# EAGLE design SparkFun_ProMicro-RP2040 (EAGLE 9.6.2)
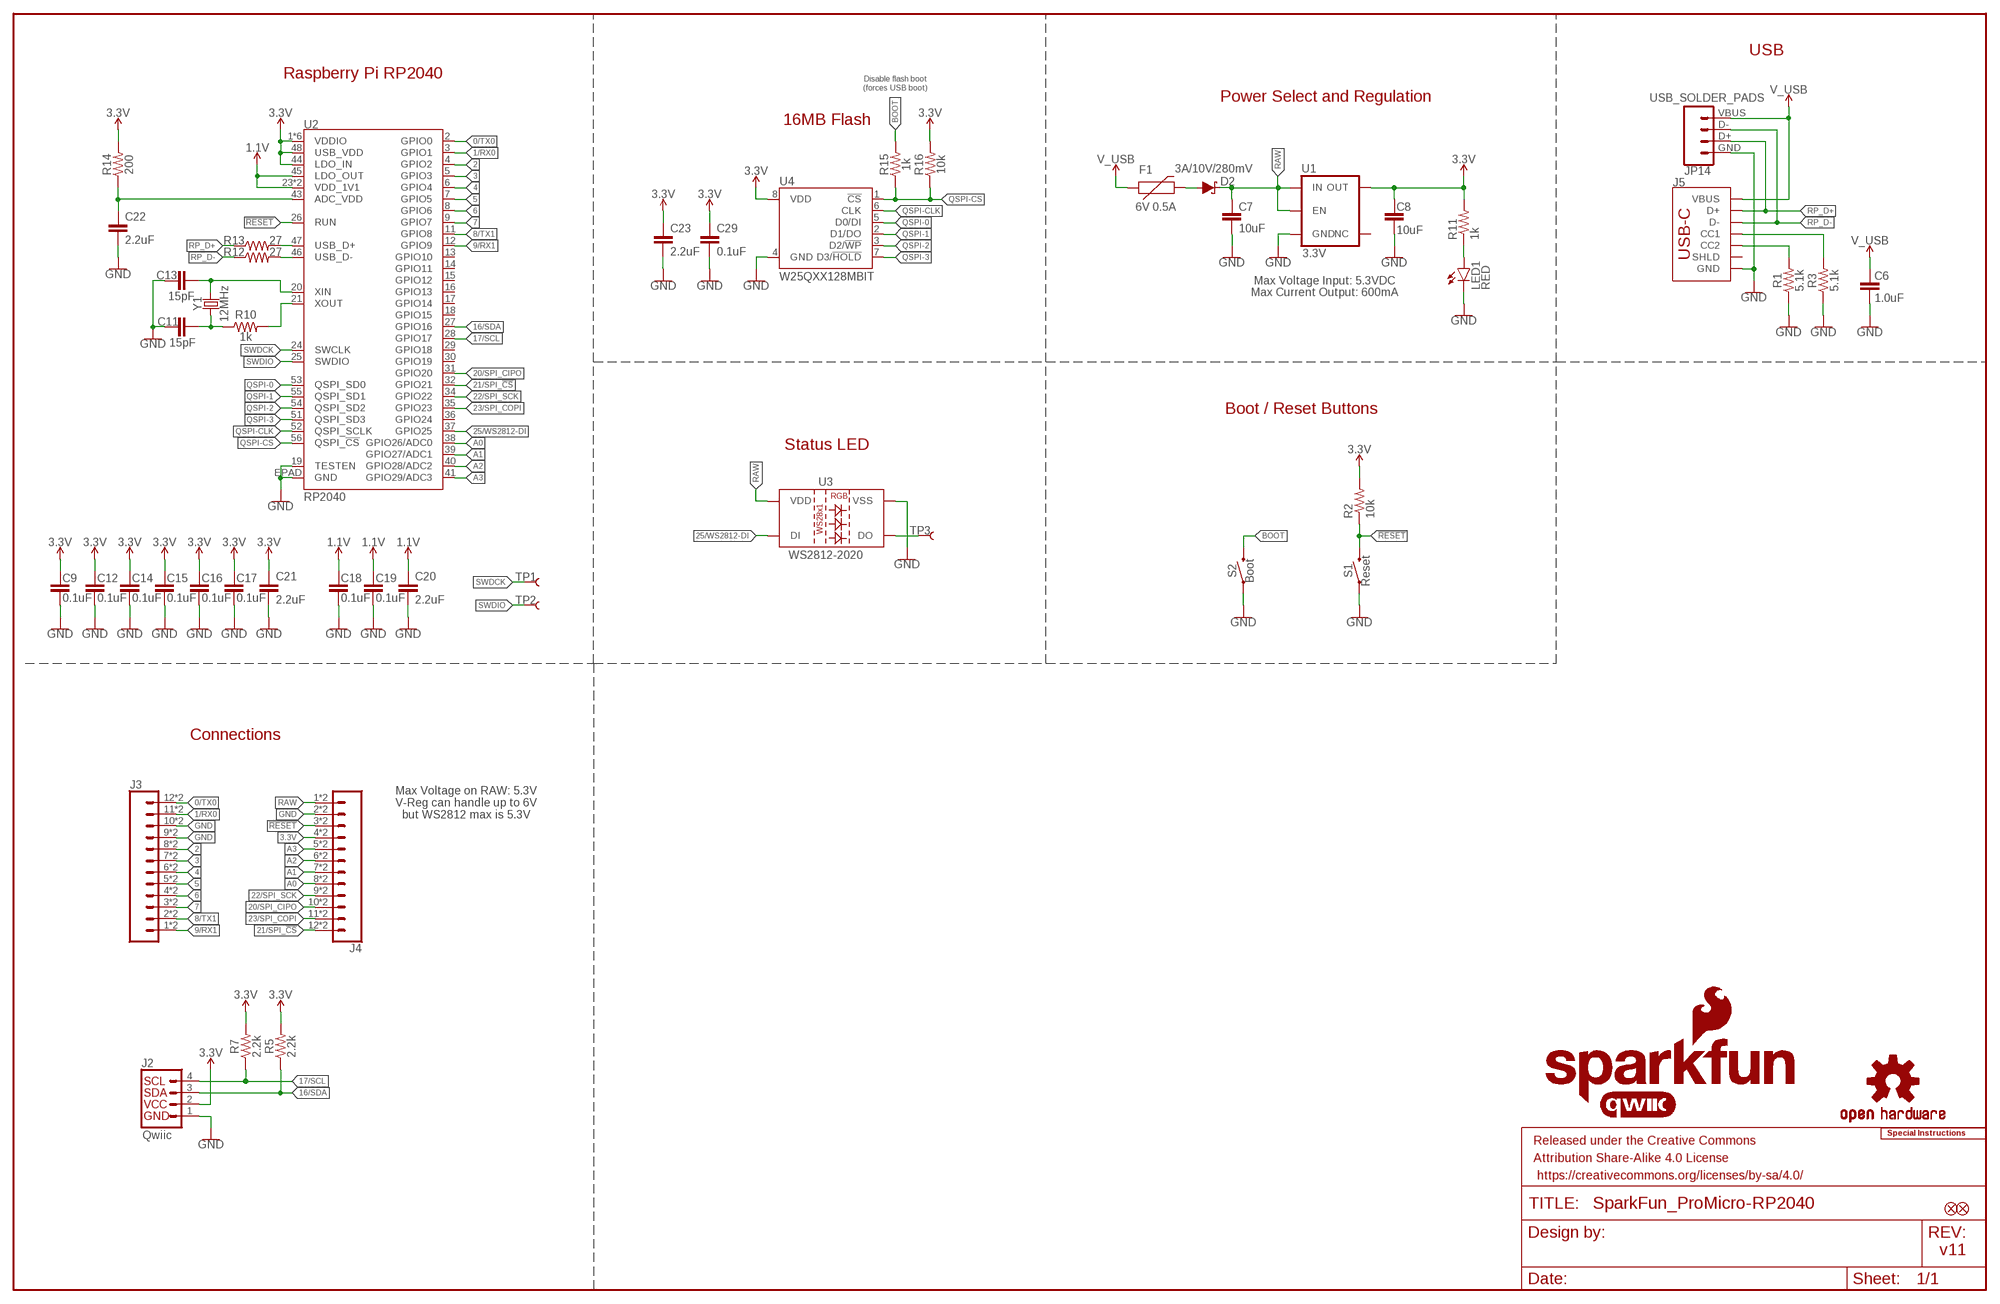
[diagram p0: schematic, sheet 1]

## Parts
C6  1.0uF  1.0UF-0402T-16V-10%  [0402-TIGHT]
C7  10uF  10UF-0402T-6.3V-20%  [0402-TIGHT]
C8  10uF  10UF-0402T-6.3V-20%  [0402-TIGHT]
C9  0.1uF  0.1UF-0402T-6.3V-10%-X7R  [0402-TIGHT]
C11  15pF  15PF-0402T-50V-5%  [0402-TIGHT]
C12  0.1uF  0.1UF-0402T-6.3V-10%-X7R  [0402-TIGHT]
C13  15pF  15PF-0402T-50V-5%  [0402-TIGHT]
C14  0.1uF  0.1UF-0402T-6.3V-10%-X7R  [0402-TIGHT]
C15  0.1uF  0.1UF-0402T-6.3V-10%-X7R  [0402-TIGHT]
C16  0.1uF  0.1UF-0402T-6.3V-10%-X7R  [0402-TIGHT]
C17  0.1uF  0.1UF-0402T-6.3V-10%-X7R  [0402-TIGHT]
C18  0.1uF  0.1UF-0402T-6.3V-10%-X7R  [0402-TIGHT]
C19  0.1uF  0.1UF-0402T-6.3V-10%-X7R  [0402-TIGHT]
C20  2.2uF  2.2UF-0402_TIGHT-10V-10%-X5R  [0402-TIGHT]
C21  2.2uF  2.2UF-0402_TIGHT-10V-10%-X5R  [0402-TIGHT]
C22  2.2uF  2.2UF-0402_TIGHT-10V-10%-X5R  [0402-TIGHT]
C23  2.2uF  2.2UF-0402_TIGHT-10V-10%-X5R  [0402-TIGHT]
C29  0.1uF  0.1UF-0402T-6.3V-10%-X7R  [0402-TIGHT]
D2  3A/10V/280mV  DIODE-SCHOTTKY-BAT60A  [SOD-323]
F1  6V 0.5A  PPTC_6V500MA  [0805]
FRAME2  FRAME-LEDGER  [CREATIVE_COMMONS]
J2  Qwiic  QWIIC_CONNECTORJS-1MM  [JST04_1MM_RA]
J3  CONN_12CASTLE  [1X12_CASTELLATED]
J4  CONN_12CASTLE  [1X12_CASTELLATED]
J5  USB Female Type C Connector  USB_C_4-LAYER_PADS  [USB-C-16P_4LAYER-PADS]
JP1  FIDUCIAL1X2  [FIDUCIAL-1X2]
JP2  FIDUCIAL1X2  [FIDUCIAL-1X2]
JP14  USB_SOLDER_PADS  [USB-SOLDER-PADS]
LED1  RED  LED-RED0603  [LED-0603]
LOGO1  SFE_LOGO_NAME_FLAME.1_INCH  [SFE_LOGO_NAME_FLAME_.1]
LOGO3  QWIIC_LOGO_6MM  [QWIIC_6MM]
LOGO4  SFE_LOGO_FLAME.1_INCH  [SFE_LOGO_FLAME_.1]
LOGO5  SPECIAL_INSTRUCTIONS-ORDERING  [ORDERING_INSTRUCTIONS]
R1  5.1k  5.1KOHM-0402T-1/16W-1%  [0402-TIGHT]
R2  10k  10KOHM-0402T-1/16W-1%  [0402-TIGHT]
R3  5.1k  5.1KOHM-0402T-1/16W-1%  [0402-TIGHT]
R5  2.2k  2.2KOHM-0402T-1/16W-1%  [0402-TIGHT]
R7  2.2k  2.2KOHM-0402T-1/16W-1%  [0402-TIGHT]
R10  1k  1KOHM-0402T-1/16W-1%  [0402-TIGHT]
R11  1k  1KOHM-0402T-1/16W-1%  [0402-TIGHT]
R12  27  27OHM  [0402-TIGHT]
R13  27  27OHM  [0402-TIGHT]
R14  200  200OHM-0402T-1/16W-1%  [0402-TIGHT]
R15  1k  1KOHM-0402T-1/16W-1%  [0402-TIGHT]
R16  10k  10KOHM-0402T-1/16W-1%  [0402-TIGHT]
S1  Reset  MOMENTARY-SWITCH-SPST-SMD-4.6X2.8MM  [TACTILE_SWITCH_SMD_4.6X2.8MM]
S2  Boot  MOMENTARY-SWITCH-SPST-SMD-4.6X2.8MM  [TACTILE_SWITCH_SMD_4.6X2.8MM]
TP1  TEST-POINT3X5  [PAD.03X.05]
TP2  TEST-POINT3X5  [PAD.03X.05]
TP3  TEST-POINT3X5  [PAD.03X.05]
U1  3.3V  V_REG_AP2112K-3.3V  [SOT23-5]
U2  RP2040  [QFN-56]
U3  WS2812-2020  [WS2812-2020]
U4  W25QXX128MBIT  W25QXX128MBIT-6X5-SKINNY_CENTER  [WSON-8-6X5-SKINNY_CENTERPAD]
U$3  OSHW-LOGOMINI  [OSHW-LOGO-MINI]
Y1  12MHz  CRYSTAL-12MHZ  [CRYSTAL-SMD-2X2.5MM]

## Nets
0/TX0: J3.12 J3.12B U2.2(GPIO0)
1.1V: C18.1 C19.1 C20.1 U2.23(VDD_1V1) U2.45(LDO_OUT) U2.50(VDD_1V1)
1/RX0: J3.11 J3.11B U2.3(GPIO1)
2: J3.8 J3.8B U2.4(GPIO2)
3: J3.7 J3.7B U2.5(GPIO3)
3.3V: C8.2 C9.1 C12.1 C14.1 C15.1 C16.1 C17.1 C21.1 C23.1 C29.1 J2.2 J4.4 J4.4B R2.2 R5.2 R7.2 R11.2 R14.2 R16.2 U1.5(OUT) U2.1(VDDIO) U2.10(VDDIO) U2.22(VDDIO) U2.33(VDDIO) U2.42(VDDIO) U2.44(LDO_IN) U2.48(USB_VDD) U2.49(VDDIO) U4.8(VDD)
4: J3.6 J3.6B U2.6(GPIO4)
5: J3.5 J3.5B U2.7(GPIO5)
6: J3.4 J3.4B U2.8(GPIO6)
7: J3.3 J3.3B U2.9(GPIO7)
8/TX1: J3.2 J3.2B U2.11(GPIO8)
9/RX1: J3.1 J3.1B U2.12(GPIO9)
16/SDA: J2.3 R5.1 U2.27(GPIO16)
17/SCL: J2.4 R7.1 U2.28(GPIO17)
20/SPI_CIPO: J4.10 J4.10B U2.31(GPIO20)
21/SPI_!CS!: J4.12 J4.12B U2.32(GPIO21)
22/SPI_SCK: J4.9 J4.9B U2.34(GPIO22)
23/SPI_COPI: J4.11 J4.11B U2.35(GPIO23)
25/WS2812-DI: U2.37(GPIO25) U3.3(DI)
!RESET!: J4.3 J4.3B R2.1 S1.3 S1.4 U2.26(RUN)
A0: J4.8 J4.8B U2.38(GPIO26/ADC0)
A1: J4.7 J4.7B U2.39(GPIO27/ADC1)
A2: J4.6 J4.6B U2.40(GPIO28/ADC2)
A3: J4.5 J4.5B U2.41(GPIO29/ADC3)
ADC_VDD: C22.1 R14.1 U2.43(ADC_VDD)
BOOT: R15.2 S2.3 S2.4
GND: C6.1 C7.1 C8.1 C9.2 C11.1 C12.2 C13.1 C14.2 C15.2 C16.2 C17.2 C18.2 C19.2 C20.2 C21.2 C22.2 C23.2 C29.2 J2.1 J3.9 J3.9B J3.10 J3.10B J4.2 J4.2B J5.GND J5.GND2(GND) JP14.GND LED1.C R1.1 R3.1 S1.1 S1.2 S2.1 S2.2 U1.2(GND) U2.19(TESTEN) U2.EPAD(GND) U3.2(VSS) U4.4(GND)
N$1: TP3.P$1 U3.1(DO)
N$9: J5.A5(CC1) R3.2
N$10: J5.B5(CC2) R1.2
N$38: LED1.A R11.1
QSPI-0: U2.53(QSPI_SD0) U4.5(D0/DI)
QSPI-1: U2.55(QSPI_SD1) U4.2(D1/DO)
QSPI-2: U2.54(QSPI_SD2) U4.3(D2/!WP!)
QSPI-3: U2.51(QSPI_SD3) U4.7(D3/!HOLD!)
QSPI-CLK: U2.52(QSPI_SCLK) U4.6(CLK)
QSPI-CS: R15.1 R16.1 U2.56(QSPI_!CS!) U4.1(!CS!)
RAW [Power]: C7.2 D2.C J4.1 J4.1B U1.1(IN) U1.3(EN) U3.4(VDD)
RP_D1+: R13.2 U2.47(USB_D+)
RP_D1-: R12.2 U2.46(USB_D-)
RP_D+: J5.A6(D+) J5.B6(D+) JP14.D+ R13.1
RP_D-: J5.A7(D-) J5.B7(D-) JP14.D- R12.1
SWDCK: TP1.P$1 U2.24(SWCLK)
SWDIO: TP2.P$1 U2.25(SWDIO)
USB_RAW [Power]: D2.A F1.2
V_USB [Power]: C6.2 F1.1 J5.VBUS1(VBUS) J5.VBUS2(VBUS) JP14.VBUS
X1A: R10.2 U2.21(XOUT)
X1B: C11.2 R10.1 Y1.P1
X2: C13.2 U2.20(XIN) Y1.P3
Unconnected: J5.SHLD1(SHLD) J5.SHLD2(SHLD) J5.SHLD3(SHLD) J5.SHLD4(SHLD) U1.4(NC) U2.13(GPIO10) U2.14(GPIO11) U2.15(GPIO12) U2.16(GPIO13) U2.17(GPIO14) U2.18(GPIO15) U2.29(GPIO18) U2.30(GPIO19) U2.36(GPIO24)

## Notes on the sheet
- USB
- Raspberry Pi RP2040
- Disable flash boot
  (forces USB boot)
- Power Select and Regulation
- 16MB Flash
- Max Voltage Input: 5.3VDC
- Max Current Output: 600mA
- Boot / Reset Buttons
- Status LED
- Connections
- Max Voltage on RAW: 5.3V
  V-Reg can handle up to 6V
  but WS2812 max is 5.3V
- v11

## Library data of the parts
C6 = SparkFun-Capacitors:1.0UF: 1µF ceramic capacitors; PROD_ID: CAP-12417
C7 C8 = SparkFun-Capacitors:10UF: 10.0µF ceramic capacitors; PROD_ID: CAP-14848
C9 C12 C14-C19 C29 = SparkFun-Capacitors:0.1UF: 0.1µF ceramic capacitors; PROD_ID: CAP-14993
C11 C13 = SparkFun-Capacitors:15PF: 15pF ceramic capacitors; PROD_ID: CAP-13063
C20-C23 = SparkFun-Capacitors:2.2UF: 2.2µF ceramic capacitors; PROD_ID: CAP-14232
D2 = SparkFun-DiscreteSemi:DIODE-SCHOTTKY: Schottky diode; PROD_ID: DIO-14072
F1 = SparkFun-Fuses:PPTC: Resettable Fuse PPTC; PROD_ID: RES-13945
FRAME2 = SparkFun-Aesthetics:FRAME-LEDGER: Schematic Frame - Ledger
J2 = SparkFun-Connectors:QWIIC_CONNECTOR: SparkFun I2C Standard Qwiic Connector An SMD 1mm pitch JST connector makes it easy and quick (get it? Qwiic?) to connect I2C devices to each other. The Qwiic system enables fast and solderless connection between popular platforms and various sensors and actuators. We carry 200mm, 100mm, 50mm, and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; PROD_ID: CONN-13694; VALUE: QWIIC_RIGHT_ANGLE
J3 J4 = Castellated:CONN_12: Multi connection point. Often used as Generic Header-pin footprint for 0.1 inch spaced/style header connections On any of the 0.1 inch spaced packages, you can populate with these: Break Away Headers - Straight (PRT-00116) Break Away Male Headers - Right Angle (PRT-00553) Female Headers (PRT-00115)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
J5 = SparkFun-Connectors:USB_C: USB Type C 16Pin Connector Super Speed pins not available on the 16-pin purely SMD connector so this part is best for USB 2.0 implementations. D1 and D2 are tied together enabling D+/- no matter which way the cable is plugged into the connector. The two channel configuration pins (CC1/2) are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; PROD_ID: CONN-14122
JP1 JP2 = SparkFun-Aesthetics:FIDUCIAL: Fiducial Alignment Points
JP14 = SparkFun-Connectors:USB_SOLDER_PADS: Solder pad access to USB pins. Helpful to expose on PCBs so user can attach external USB connector if necessary.
LED1 = SparkFun-LED:LED-RED: Red SMD LED; PROD_ID: DIO-00819
LOGO1 = SparkFun-Aesthetics:SFE_LOGO_NAME_FLAME: SparkFun Font Logo w/ Flame
LOGO3 = SparkFun-Aesthetics:QWIIC_LOGO: Qwiic Logos for placement on schematic and PCB. The 5.5mm silk logo is best for placing next to Qwiic connector.
LOGO4 = SparkFun-Aesthetics:SFE_LOGO_FLAME: SparkFun Flame Logo
LOGO5 = SparkFun-Aesthetics:SPECIAL_INSTRUCTIONS: Special Ordering/Production Instructions Alert
R1 R3 = SparkFun-Resistors:5.1KOHM; PROD_ID: RES-14340
R2 R16 = SparkFun-Resistors:10KOHM: 10kΩ resistor; PROD_ID: RES-14241
R5 R7 = SparkFun-Resistors:2.2KOHM: 2.2kΩ resistor; PROD_ID: RES-14341
R10 R11 R15 = SparkFun-Resistors:1KOHM: 1kΩ resistor; PROD_ID: RES-14342
R12 R13 = SparkFun-Resistors:27OHM: 27Ω resistor; PROD_ID: RES-15238
R14 = SparkFun-Resistors:200OHM: 200Ω resistor; PROD_ID: RES-15550
S1 S2 = SparkFun-Switches:MOMENTARY-SWITCH-SPST: Momentary Switch (Pushbutton) - SPST; PROD_ID: SWCH-15606
TP1-TP3 = SparkFun-Connectors:TEST-POINT: SparkFun Test Points
U1 = SparkFun-IC-Power:V_REG_AP2112: AP2112 - 600mA CMOS LDO Regulator w/ Enable The AP2112 is CMOS process low dropout linear regulator with enable function, the regulator delivers a guaranteed 600mA (min.) continuous load current. Features Output Voltage Accuracy: ±1.5% Output Current: 600mA (Min.) Foldback Short Current Protection: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; PROD_ID: VREG-12457
U2 = RP2040:RP2040: Raspberry Pi RP2040 MCU 56-pin 32-bit Microcontroller with 264kB of SRAM and external flash support up to 16MB Getting Started with the RP2040 Dual-core ARM Cortex M0+ processor, flexible clock running up to 133 MHz 264kB of SRAM, and QSPI control of common flash memory USB 1.1 Host and Device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; PROD_ID: IC-15502
U3 = SparkFun-LED:WS2812-2020; PROD_ID: DIO-15591
U4 = SparkFun-IC-Memory:W25QXX; PROD_ID: IC-15107
U$3 = SparkFun-Aesthetics:OSHW-LOGO: Open-Source Hardware (OSHW) Logo
Y1 = SparkFun-Clocks:CRYSTAL-12MHZ: 12.0MHz Crystal; PROD_ID: XTAL-15540

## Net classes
1 Power: width 0.127 mm, clearance 0.178 mm

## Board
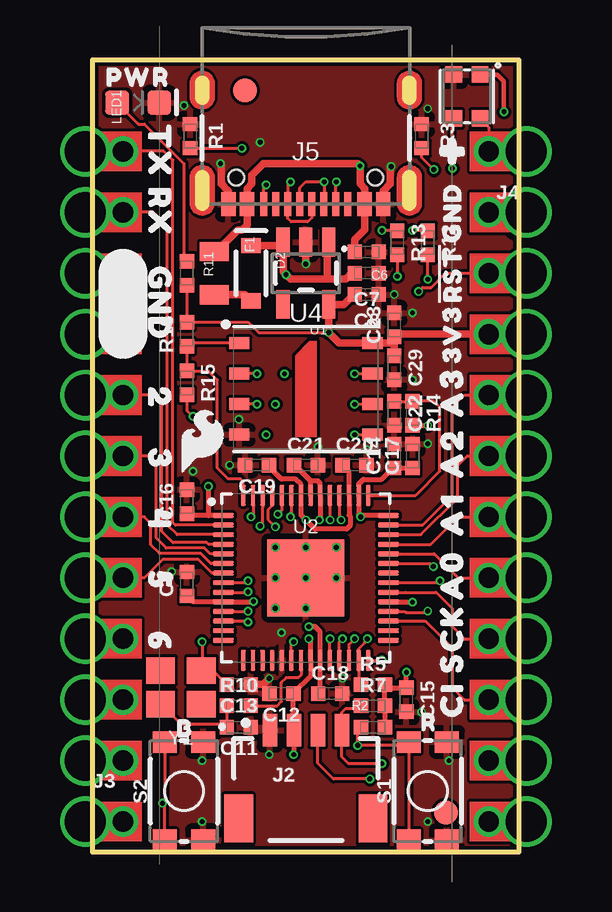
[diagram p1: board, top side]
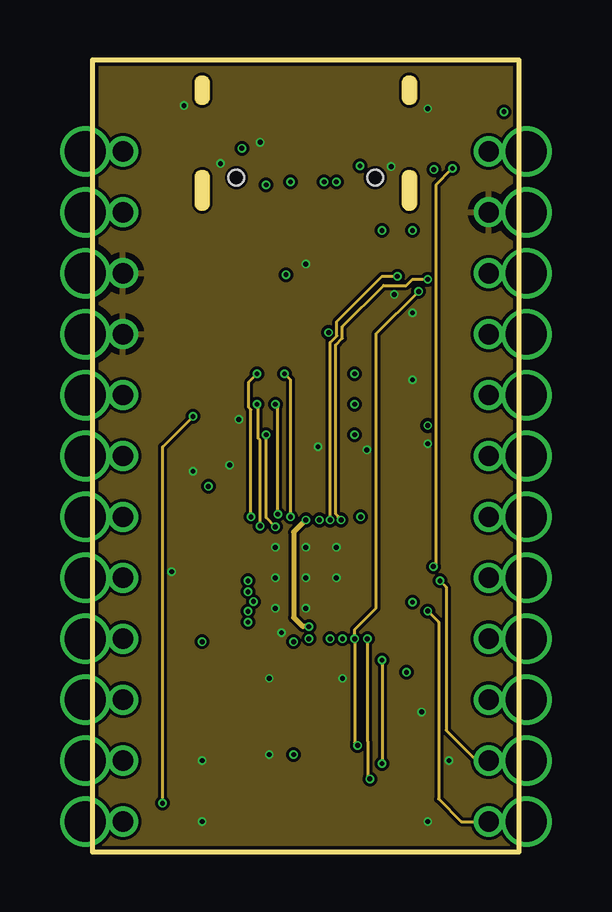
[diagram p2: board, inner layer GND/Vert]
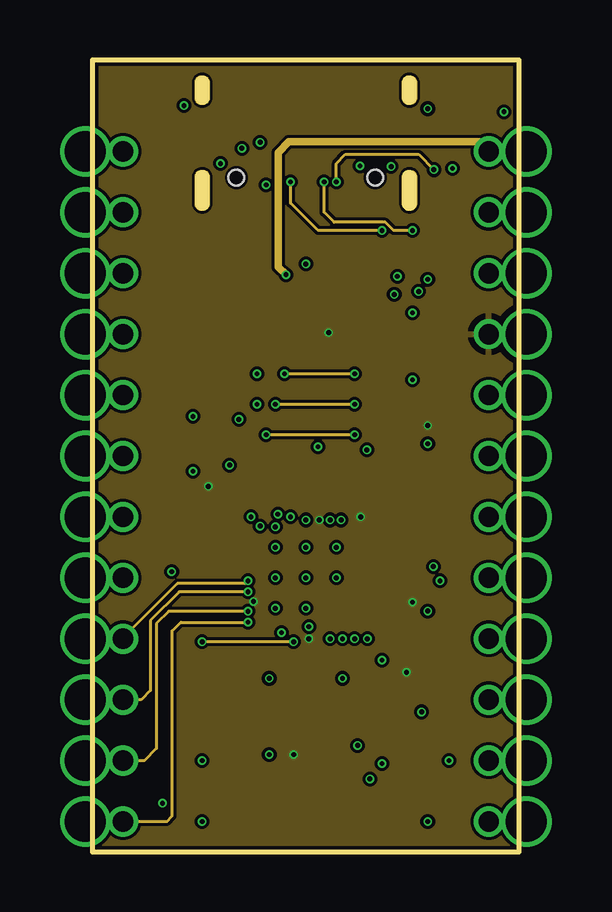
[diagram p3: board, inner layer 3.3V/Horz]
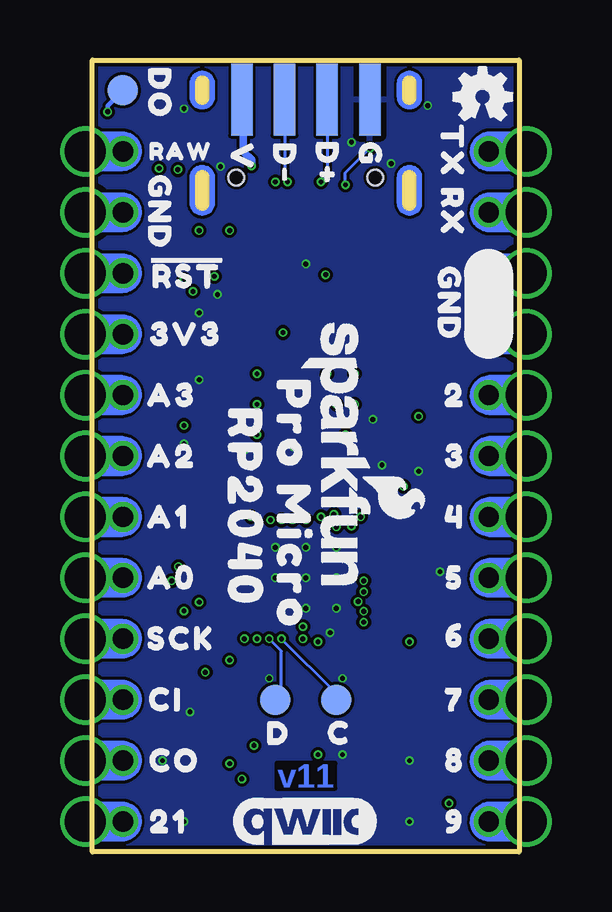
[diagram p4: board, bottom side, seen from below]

Size 17.78 x 33.02 mm. Coordinates in mm from the lower left corner, seen from the top.
Outline: 0,33.02 0,0 17.78,0 17.78,33.02 0,33.02
Copper layers (1+2*15+16): Top 0.035mm / dielectric 1.5mm / GND/Vert 0.035mm / dielectric 0.15mm / 3.3V/Horz 0.035mm / dielectric 0.2mm / Bottom 0.035mm
Design rules "SparkFun-4-layer-MicroMod *": minimum track width 4mil, minimum drill 0.2mm, track to track 4mil, track to pad 4mil, pad to pad 4mil, via to via 4mil, smd to smd 4mil, copper to edge 6mil, drill to drill 6mil, minimum pad ring 3mil, minimum via ring 3mil, stop-mask expansion 4mil, vias tented up to drill 25mil, thermal gap 10mil

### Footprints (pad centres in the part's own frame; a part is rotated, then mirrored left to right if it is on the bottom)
0402-TIGHT = smd 0.6 x 0.6: 1 -0.5,0; 2 0.5,0
SOD-323 = smd 0.63 x 0.83: A 1.15,0; C -1.15,0
0805 = smd 0.8 x 1.2: 1 -0.9,0; 2 0.9,0
JST04_1MM_RA = smd 0.6 x 1.35: 1 -1.5,0; 2 -0.5,0; 3 0.5,0; 4 1.5,0 | smd 1.2 x 2: NC1 2.8,-3.675; NC2 -2.8,-3.675
1X12_CASTELLATED = drill 0.85 pad 1.016: 1 0,0; 2 0,2.54; 3 0,5.08; 4 0,7.62; 5 0,10.16; 6 0,12.7; 7 0,15.24; 8 0,17.78; 9 0,20.32; 10 0,22.86; 11 0,25.4; 12 0,27.94 | drill 1.7 pad 1.75: 1B -1.57,0; 2B -1.57,2.54; 3B -1.57,5.08; 4B -1.57,7.62; 5B -1.57,10.16; 6B -1.57,12.7; 7B -1.57,15.24; 8B -1.57,17.78; 9B -1.57,20.32; 10B -1.57,22.86; 11B -1.57,25.4; 12B -1.57,27.94
USB-C-16P_4LAYER-PADS = smd 0.3 x 1: A5 -1.25,-0.34; A6 -0.25,-0.34; A7 0.25,-0.34; A8 1.25,-0.34; B5 1.75,-0.34; B6 0.75,-0.34; B7 -0.75,-0.34; B8 -1.75,-0.34 | smd 0.6 x 1: GND -3.225,-0.34; GND2 3.225,-0.34; VBUS1 -2.45,-0.34; VBUS2 2.45,-0.34 | drill 0.4 pad 0.6 long: SHLD1 -4.318,-0.915; SHLD2 4.318,-0.915; SHLD3 -4.318,-5.095; SHLD4 4.318,-5.095 | hole 0.65: -2.89,-1.445; 2.89,-1.445
FIDUCIAL-1X2 = smd 1 x 1: 1 0,0
USB-SOLDER-PADS = smd 3 x 0.9: D+ 0,-0.889; D- 0,0.889; GND 0,-2.667; VBUS 0,2.667
LED-0603 = smd 1 x 1: A -0.877,0; C 0.877,0
TACTILE_SWITCH_SMD_4.6X2.8MM = smd 0.9 x 1: 1 -2.05,-0.8; 2 2.05,-0.8; 3 2.05,0.8; 4 -2.05,0.8
PAD.03X.05 = smd 1.27 x 1.27: P$1 0,0
SOT23-5 = smd 0.55 x 1.2: 1 -0.95,-1.3; 2 0,-1.3; 3 0.95,-1.3; 4 0.95,1.3; 5 -0.95,1.3
QFN-56 = smd 0.875 x 0.2: 1 -3.437,2.6; 2 -3.437,2.2; 3 -3.437,1.8; 4 -3.437,1.4; 5 -3.437,1; 6 -3.437,0.6; 7 -3.437,0.2; 8 -3.437,-0.2; 9 -3.437,-0.6; 10 -3.437,-1; 11 -3.437,-1.4; 12 -3.437,-1.8; 13 -3.437,-2.2; 14 -3.437,-2.6; 29 3.437,-2.6; 30 3.437,-2.2; 31 3.437,-1.8; 32 3.437,-1.4; 33 3.437,-1; 34 3.437,-0.6; 35 3.437,-0.2; 36 3.437,0.2; 37 3.437,0.6; 38 3.437,1; 39 3.437,1.4; 40 3.437,1.8; 41 3.437,2.2; 42 3.437,2.6 | smd 0.2 x 0.875: 15 -2.6,-3.437; 16 -2.2,-3.437; 17 -1.8,-3.437; 18 -1.4,-3.437; 19 -1,-3.437; 20 -0.6,-3.437; 21 -0.2,-3.437; 22 0.2,-3.437; 23 0.6,-3.437; 24 1,-3.437; 25 1.4,-3.437; 26 1.8,-3.437; 27 2.2,-3.437; 28 2.6,-3.437; 43 2.6,3.437; 44 2.2,3.437; 45 1.8,3.437; 46 1.4,3.437; 47 1,3.437; 48 0.6,3.437; 49 0.2,3.437; 50 -0.2,3.437; 51 -0.6,3.437; 52 -1,3.437; 53 -1.4,3.437; 54 -1.8,3.437; 55 -2.2,3.437; 56 -2.6,3.437 | smd 3.2 x 3.2: EPAD 0,0
WS2812-2020 = smd 0.7 x 0.7: 1 0.915,-0.55; 2 0.915,0.55; 3 -0.915,0.55; 4 -0.915,-0.55
WSON-8-6X5-SKINNY_CENTERPAD = smd 0.85 x 0.5: 1 -2.775,1.905; 2 -2.775,0.635; 3 -2.775,-0.635; 4 -2.775,-1.905; 5 2.775,-1.905; 6 2.775,-0.635; 7 2.775,0.635; 8 2.775,1.905
CRYSTAL-SMD-2X2.5MM = smd 1.2 x 1.1: P1 0.846,0.69; P2 -0.854,0.69; P3 -0.854,-0.71; P4 0.846,-0.71

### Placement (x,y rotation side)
C6  11.43,25.02 180 top
C7  11.43,24.13 180 top
C8  11.43,23.24 180 top
C9  3.94,11.18 90 top
C11  6.1,5.21 180 top
C12  7.87,6.6 180 top
C13  6.1,6.99 180 top
C14  12.57,16.51 90 top
C15  13.08,6.35 270 top
C16  3.94,14.61 90 top
C17  13.34,16.51 90 top
C18  9.91,6.6 0 top
C19  6.86,16.13 180 top
C20  10.92,16.13 0 top
C21  8.89,16.13 0 top
C22  12.57,18.29 270 top
C23  12.57,21.97 90 top
C29  12.57,20.19 270 top
D2  6.6,24.13 270 top
F1  5.08,24.13 270 top
FRAME2  not placed on the board
J2  8.89,5.08 0 top
J3  1.27,1.27 0 top
J4  16.51,29.21 180 top
J5  8.89,26.67 180 top
JP1  14.73,1.65 0 top
JP2  6.35,31.75 0 top
JP14  8.89,31.37 90 bottom
LED1  1.91,31.24 0 top
LOGO1  7.62,16.51 270 bottom
LOGO3  8.89,1.27 0 bottom
LOGO4  4.57,17.14 0 top
LOGO5  not placed on the board
R1  4.06,29.84 270 top
R2  11.68,5.21 0 top
R3  13.72,29.84 270 top
R5  11.68,6.99 0 top
R7  11.68,6.1 0 top
R10  6.1,6.1 0 top
R11  3.94,24.13 270 top
R12  13.97,25.4 270 top
R13  12.7,25.4 270 top
R14  13.34,18.29 270 top
R15  3.94,19.56 270 top
R16  3.94,21.59 90 top
S1  13.97,2.54 90 top
S2  3.81,2.54 90 top
TP1  7.62,6.35 0 bottom
TP2  10.16,6.35 0 bottom
TP3  16.51,31.75 0 bottom
U1  8.89,24.13 180 top
U2  8.89,11.43 0 top
U3  15.6,31.5 90 top
U4  8.89,19.3 0 top
U$1  [A00]  14.99,11.56 90 top
U$2  [GND_0]  14.99,26.8 90 top
U$3  1.52,31.5 0 bottom
U$4  [PRO_MICRO0]  9.4,14.48 270 bottom
U$5  [#0]  15.1,29.2 0 top
U$6  [70]  2.67,6.35 0 bottom
U$7  [81]  2.67,3.81 0 bottom
U$8  [92]  2.67,1.27 0 bottom
U$9  [CI4]  14.73,6.35 0 bottom
U$10  [SCK3]  14.1,8.89 0 bottom
U$11  [A00]  14.48,11.43 0 bottom
U$12  [A10]  14.61,13.97 0 bottom
U$13  [A21]  14.48,16.51 0 bottom
U$14  [A32]  14.48,19.05 0 bottom
U$15  [GND2]  14.99,26.67 270 bottom
U$16  [3V3_0]  13.72,21.59 0 bottom
U$17  [RAW0]  14.1,29.21 0 bottom
U$18  [C0]  7.49,4.95 0 bottom
U$19  [TX0]  2.79,29.21 270 bottom
U$20  [A10]  14.99,14.1 90 top
U$21  [RX1]  2.79,26.67 270 bottom
U$22  [GND2]  2.92,22.86 270 bottom
U$23  [20]  2.67,19.05 0 bottom
U$24  [31]  2.67,16.51 0 bottom
U$25  [42]  2.67,13.97 0 bottom
U$26  [53]  2.67,11.43 0 bottom
U$27  [64]  2.67,9.02 0 bottom
U$28  [D#1]  8,28.7 270 bottom
U$29  [D#2]  9.78,28.7 270 bottom
U$30  [G0]  6.22,29.08 270 bottom
U$31  [V3]  11.56,28.96 270 bottom
U$32  [210]  14.61,1.27 0 bottom
U$33  [A21]  14.99,16.64 90 top
U$34  [#RST#0]  13.84,24.13 0 bottom
U$35  [D1]  10.03,4.95 0 bottom
U$36  [B0]  3.86,5.16 0 top
U$37  [R0]  14.02,5.41 0 top
U$38  [RP20401]  11.43,14.35 270 bottom
U$39  [A32]  14.99,19.18 90 top
U$40  [DO0]  14.99,31.62 270 bottom
U$53  [20]  2.79,18.92 270 top
U$54  [31]  2.79,16.38 270 top
U$55  [42]  2.79,13.84 270 top
U$56  [53]  2.79,11.3 270 top
U$57  [64]  2.79,8.76 270 top
U$64  [CI4]  14.99,6.35 90 top
U$66  [CO5]  14.35,3.81 0 bottom
U$67  [SCK3]  14.99,8.89 90 top
U$68  [#RST#1]  14.9,24.1 90 top
U$69  [3V30]  14.99,21.59 90 top
U$73  [PWR0]  1.9,32.3 0 top
U$74  [GND2]  2.79,22.86 270 top
U$75  [RX1]  2.79,26.67 270 top
U$76  [TX0]  2.79,29.21 270 top
Y1  3.68,6.86 180 top

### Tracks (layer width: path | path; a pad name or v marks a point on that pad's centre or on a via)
0/TX0
  Top 0.127: U2.2 3.45,13.63 3.35,13.74 3.35,28.84 2.98,29.21 J3.12
  3.3V/Horz 0.127: J3.12B J3.12
1.1V  (via drill 0.2)
  Top 0.127: 7.36,16.06 C19.1 | 9.49,6.69 C18.1
  Top 0.203: 7.36,16.06 7.87,15.54 8.46,15.54 8.69,15.31 U2.50 8.69,14.04 v8.89,13.84 9.27,13.46 10.59,13.46 10.74,13.61 10.74,14 10.69,14.05 U2.45 10.69,15.86 C20.1 | 9.49,6.69 U2.23 9.49,9.18 9.27,9.4 v9.02,9.4
  GND/Vert 0.203: v9.02,9.4 8.76,9.4 8.38,9.78 8.38,13.34 v8.89,13.84
1/RX0
  Top 0.127: J3.11 2.54,26.67 3.12,26.09 3.12,13.64 3.53,13.23 U2.3
  3.3V/Horz 0.127: J3.11B J3.11
2
  Top 0.127: U2.4 4.83,12.83 4.76,12.9 3.35,12.9 2.89,13.37 2.89,18.7 2.54,19.05 J3.8 J3.8B
3
  Top 0.127: U2.5 4.91,12.43 4.67,12.68 3.07,12.68 2.66,13.09 2.66,16.14 2.29,16.51 J3.7 J3.7B
3.3V  (via drill 0.2)
  Top 0.127: 4.01,14.03 C16.1 | R5.2 12.32,6.85 | J2.2 8.37,5.1 | 8.39,4.07 v8.38,4.06 | R11.2 R16.2 6.49,22.09 6.92,21.66 v9.84,21.66 | 10.89,23.24 C8.2 | C23.1 12.69,21.59 | J4.4B J4.4 | 8.43,16.13 C21.1 | v6.7,10.43 v6.71,10.44 | v13.96,17.79 v13.97,17.78
  Top 0.203: U2.1 4.83,14.03 | 4.83,14.03 4.01,14.03 | R5.2 R7.2 R2.2 | 12.32,6.85 C15.1 v13.08,7.49 | U2.33 13.32,10.43 v13.34,10.41 | v9.02,8.89 9.09,8.82 U2.22 9.09,7.32 C12.1 8.37,5.1 | J2.2 8.39,4.07 | C9.1 4.18,10.43 U2.10 v6.7,10.43 | U2.42 11.24,14.03 v11.18,13.97 11.09,14.06 U2.44 11.09,15.34 11.29,15.54 12.04,15.54 12.52,16.01 C14.1 C17.1 | v4.83,15.24 4.83,14.03 | R14.2 v13.96,17.79 | v9.45,13.84 9.49,13.88 U2.48 9.49,15.37 9.39,15.47 9.09,15.47 | U2.49 9.09,15.47 | 9.09,15.47 8.43,16.13
  Top 0.305: 10.89,23.24 10.47,22.83 U1.5 v9.84,21.66 10.29,21.21 U4.8 12.57,21.21 | 12.69,21.59 J4.4 | C29.1 12.57,21.21 | 12.57,21.21 C23.1
  pour 3.3V/Horz (isolate 0.127): 0,33.02 17.78,33.02 17.78,0 0,0
4
  Top 0.127: J3.6B J3.6 2.16,13.97 2.43,13.7 2.43,12.81 2.79,12.45 4.51,12.45 4.93,12.03 U2.6
5
  Top 0.127: J3.5B J3.5 2.16,11.43 2.92,12.19 4.42,12.19 4.98,11.63 U2.7
6  (via drill 0.2)
  Top 0.127: U2.8 6.4,11.23 v6.48,11.3 | J3.4B J3.4
  3.3V/Horz 0.127: v6.48,11.3 6.36,11.19 3.54,11.19 1.27,8.92 J3.4
7  (via drill 0.2)
  Top 0.127: U2.9 6.46,10.83 v6.48,10.85 | J3.3B J3.3
  3.3V/Horz 0.127: v6.48,10.85 3.61,10.85 2.41,9.65 2.41,6.73 2.03,6.35 J3.3
8/TX1  (via drill 0.2)
  Top 0.127: U2.11 v6.47,10.03 v6.48,10.03 | J3.2B J3.2
  3.3V/Horz 0.127: v6.48,10.03 3.17,10.03 2.67,9.53 2.67,4.32 2.16,3.81 J3.2
9/RX1  (via drill 0.2)
  Top 0.127: U2.12 6.43,9.63 v6.48,9.58 | J3.1B J3.1
  3.3V/Horz 0.127: J3.1 3.09,1.27 3.32,1.5 3.32,9.22 3.68,9.58 v6.48,9.58
16/SDA  (via drill 0.2)
  Top 0.127: R5.1 11.09,7.08 U2.27 11.09,8.47 11.34,8.72 11.34,8.78 v11.45,8.89 | v11.56,3.05 10.03,3.05 9.39,3.69 J2.3
  GND/Vert 0.127: v11.45,8.89 11.45,4.63 11.47,4.62 11.47,3.14 v11.56,3.05
17/SCL  (via drill 0.2)
  Top 0.127: U2.28 v12.06,7.99 v12.06,8 | v12.06,3.68 10.67,3.68 10.39,3.96 J2.4 10.39,5.82 10.54,5.97 11.06,5.97 R7.1
  GND/Vert 0.127: v12.06,8 v12.06,3.68
20/SPI_CIPO
  Top 0.127: U2.31 13.87,9.63 14.99,8.51 14.99,6.86 15.49,6.35 J4.10 J4.10B
21/SPI_!CS!  (via drill 0.2)
  Top 0.127: U2.32 13,10.03 13.04,10 13.92,10 v13.97,10.05 | J4.12B J4.12
  GND/Vert 0.127: v13.97,10.05 14.43,9.59 14.43,2.21 15.37,1.27 J4.12
22/SPI_SCK
  Top 0.127: U2.34 13.03,10.83 13.04,10.83 14.31,10.83 14.99,10.16 14.99,9.4 15.49,8.89 J4.9 J4.9B
23/SPI_COPI  (via drill 0.2)
  Top 0.127: U2.35 14.4,11.23 v14.48,11.3 | J4.11B J4.11
  GND/Vert 0.127: v14.48,11.3 14.73,11.05 14.73,5.08 16,3.81 J4.11
25/WS2812-DI  (via drill 0.2)
  Top 0.127: U2.37 14.07,12.03 v14.2,11.9 | v15,28.5 15,30.54 U3.3
  GND/Vert 0.127: v14.2,11.9 14.31,12.01 14.31,27.81 v15,28.5
!RESET!  (via drill 0.2)
  Top 0.127: U2.26 10.69,8.66 v10.92,8.89 | R2.1 11.05,5.07 v11.05,4.45 13.03,4.45 S1.3 S1.4 | J4.3B J4.3 14.71,24.13 14.11,23.54 13.76,23.54 v13.59,23.37
  GND/Vert 0.127: v11.05,4.45 10.92,4.57 v10.92,8.89 10.92,9.27 11.81,10.16 11.81,21.59 v13.59,23.37
A0
  Top 0.127: U2.38 14.24,12.43 15.24,11.43 J4.8 J4.8B
A1
  Top 0.127: U2.39 14.1,12.83 15.24,13.97 J4.7 J4.7B
A2
  Top 0.127: U2.40 13.68,13.23 15.21,14.76 15.21,16.1 15.62,16.51 J4.6 J4.6B
A3
  Top 0.127: U2.41 13.76,13.63 14.99,14.86 14.99,18.54 15.49,19.05 J4.5 J4.5B
ADC_VDD
  Top 0.127: U2.43 13.47,14.87 14.48,15.88 14.48,18.54 14.22,18.8 R14.1 C22.1
BOOT  (via drill 0.2)
  Top 0.127: S2.4 3.01,1.94 v2.92,2.03 3.01,2.12 S2.3 | R15.2 3.94,18.41 v4.19,18.16
  GND/Vert 0.127: v2.92,2.03 2.92,16.89 v4.19,18.16
GND  (via drill 0.2)
  Top 0.305: U1.2 v8.89,24.51 | J5.GND 12.12,27.56 12.41,27.85 12.41,28.54 v12.45,28.57 | J5.GND2 5.67,27.56 5.37,27.85 5.37,28.67 v5.33,28.7 | C13.1 7.11,6.99 v7.37,7.24
  other vias: 4.19,15.88 5.71,16.13 9.4,16.89 11.43,16.76 13.97,17.02 13.34,19.68 13.34,22.48 12.57,23.24 3.81,31.11 6.99,29.59 13.97,30.99 6.1,18.03 7.87,9.14 10.41,7.24 7.37,4.06 4.57,3.81 4.57,1.27 14.86,3.81 13.97,1.27 13.72,5.84 3.3,11.68 7.62,10.16 7.62,12.7 10.16,12.7 8.89,10.16 8.89,11.43 7.62,11.43 10.16,11.43 8.89,12.7
  pour Top (isolate 0.127): 0,33.02 17.78,33.02 17.78,0 0,0
  pour Bottom (isolate 0.127): 0,33.02 17.78,33.02 17.78,0 0,0
  pour GND/Vert (isolate 0.127): 0,33.02 17.78,33.02 17.78,0 0,0
N$1  (via drill 0.2)
  Top 0.178: v17.14,30.86 17.14,32.13 16.86,32.41 U3.1
  Bottom 0.178: TP3.P$1 17.14,31.11 v17.14,30.86
N$9  (via drill 0.2)
  Top 0.127: J5.A5 10.14,27.92 v10.16,27.94 | v14.22,28.45 13.72,28.96 R3.2
  3.3V/Horz 0.127: v10.16,27.94 10.16,28.7 10.54,29.08 13.59,29.08 v14.22,28.45
N$10  (via drill 0.2)
  Top 0.127: J5.B5 7.14,27.71 v7.24,27.81 | R1.2 v6.21,29.34 v6.22,29.34
  Bottom 0.127: v7.24,27.81 7.24,28.32 v6.22,29.34
N$38
  Top 0.127: R11.1 3.81,24.76 3.81,28.7 2.16,30.35 1.92,30.35 LED1.A
QSPI-0  (via drill 0.2)
  Top 0.127: U2.53 7.49,14.44 7.31,14.26 7.31,13.87 v7.62,13.56 | v10.92,17.4 U4.5
  GND/Vert 0.127: v7.62,13.56 7.24,13.94 v7.24,17.4
  3.3V/Horz 0.127: v7.24,17.4 v10.92,17.4
QSPI-1  (via drill 0.2)
  Top 0.127: U2.55 6.69,14.06 v6.6,13.97 | v6.86,19.94 U4.2
  GND/Vert 0.127: v6.6,13.97 6.6,18.44 6.52,18.53 6.52,19.6 v6.86,19.94
QSPI-2  (via drill 0.2)
  Top 0.127: U2.54 7.09,14.37 7.08,14.35 7.08,13.68 v6.99,13.59 | v6.86,18.67 U4.3
  GND/Vert 0.127: v6.99,13.59 6.99,17.17 6.9,17.26 6.9,18.63 v6.86,18.67
QSPI-3  (via drill 0.2)
  Top 0.127: U2.51 8.29,14.01 v8.26,13.97 | v10.92,19.94 U4.7
  GND/Vert 0.127: v8.26,13.97 8.26,19.68 v8,19.94
  3.3V/Horz 0.127: v8,19.94 v10.92,19.94
QSPI-CLK  (via drill 0.2)
  Top 0.127: U2.52 7.89,14.25 v7.72,14.09 | v10.92,18.67 U4.6
  GND/Vert 0.127: v7.72,14.09 7.72,18.56 v7.62,18.67
  3.3V/Horz 0.127: v7.62,18.67 v10.92,18.67
QSPI-CS
  Top 0.127: U2.56 6.29,15.43 6.16,15.55 5.66,15.55 5.21,16 5.21,19.68 4.83,20.06 R15.1 R16.1 4.06,21.21 U4.1
RAW  (via drill 0.2)
  Top 0.127: J4.1B J4.1 16.51,30.23 U3.4
  Top 0.305: D2.C 7.79,25.28 U1.3 7.94,24.19 v8.06,24.07 8.26,23.88 9.78,23.88 | C7.2 10.8,24.13 10.55,23.88 9.78,23.88 | U1.1 9.78,25.37 9.78,23.88
  3.3V/Horz 0.305: v8.06,24.07 7.75,24.38 7.75,29.16 8.19,29.6 16.12,29.6 J4.1
RP_D1+  (via drill 0.2)
  Top 0.127: U2.47 9.89,13.86 v9.91,13.84 | R13.2 v12.7,24
  GND/Vert 0.127: v12.7,24 12.06,24 10.18,22.12 10.18,21.52 9.91,21.24 v9.91,13.84
RP_D1-  (via drill 0.2)
  Top 0.127: U2.46 10.29,13.91 v10.36,13.84 | v13.97,23.88 R12.2
  GND/Vert 0.127: v10.36,13.84 10.25,13.96 10.25,13.98 10.13,14.1 10.13,21.14 10.41,21.42 10.41,21.9 12.13,23.62 13.08,23.62 13.34,23.88 v13.97,23.88
RP_D+  (via drill 0.2)
  Top 0.127: R13.1 12.07,25.9 v12.06,25.91 | v8.26,27.94 8.14,27.82 J5.B6 8.13,27 8.13,26.42 8.27,26.27 8.97,26.27 9.14,26.45 J5.A6
  3.3V/Horz 0.127: v12.06,25.91 9.4,25.91 8.26,27.05 v8.26,27.94
  Bottom 0.127: JP14.D+ 8,28.19 v8.26,27.94
RP_D-  (via drill 0.2)
  Top 0.127: R12.1 v13.34,25.9 v13.34,25.91 | J5.B7 9.65,27.02 v9.65,27.94 8.89,27.94 8.64,27.69 J5.A7
  3.3V/Horz 0.127: v13.34,25.91 12.55,25.91 12.21,26.25 10.07,26.25 9.65,26.67 v9.65,27.94
  Bottom 0.127: JP14.D- 9.78,28.07 v9.65,27.94
SWDCK  (via drill 0.2)
  Top 0.127: U2.24 9.89,8.87 v9.91,8.89
  Bottom 0.127: TP1.P$1 7.62,6.6 v9.91,8.89
SWDIO  (via drill 0.2)
  Top 0.127: U2.25 10.29,8.77 v10.41,8.89
  Bottom 0.127: TP2.P$1 10.16,6.6 9.91,6.86 9.91,8.38 v10.41,8.89
USB_RAW
  Top 0.305: F1.2 6.35,23.23 D2.A
V_USB  (via drill 0.2)
  Top 0.305: F1.1 5.16,25.03 6.05,25.93 6.22,25.93 6.44,26.14 J5.VBUS2 6.44,27.66 6.63,27.85 6.63,28.22 7.11,28.7 11.05,28.7 v11.15,28.6 11.15,27.85 11.34,27.66 J5.VBUS1 11.34,25.95 10.93,25.54 C6.2
  Bottom 0.305: v11.15,28.6 11.15,28.86 11.49,29.2 11.49,31.3 JP14.VBUS
X1A
  Top 0.127: U2.21 8.69,7.39 8.56,7.26 8.07,7.26 7.87,7.06 7.87,6.27 7.7,6.1 R10.2
X1B
  Top 0.127: Y1.P1 3.68,5.33 5.6,5.33 | R10.1 5.6,5.33 | 5.6,5.33 C11.2
X2  (via drill 0.2)
  Top 0.127: U2.20 8.29,8.67 v8.38,8.76 | v4.57,8.76 4.57,7.6 Y1.P3 5.01,7.57 C13.2
  3.3V/Horz 0.127: v8.38,8.76 v4.57,8.76

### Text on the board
Bottom: v11
Measures: Units in Inches
tDocu: 0.8mm PCB | N Seidle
